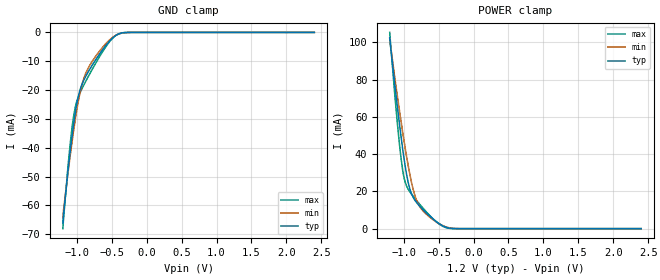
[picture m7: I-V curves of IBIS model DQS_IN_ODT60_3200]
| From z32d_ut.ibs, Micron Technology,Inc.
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| MODEL DQS_IN_ODT60_3200 (Data Strobe Input with 60ohm ODT, 1600-3200Mbps)
[Model]   DQS_IN_ODT60_3200
Model_type   Input
Vinl = 905.000mV
Vinh = 1015.000mV
|   typ   min   max
|C_comp   0.596pF   0.538pF   0.646pF
C_comp_power_clamp   0.298pF   0.269pF   0.323pF
C_comp_gnd_clamp   0.298pF   0.269pF   0.323pF
| Note: C_comp changes when the ODT circuit is enabled.
|[Model Spec]
| Dynamic Overshoot Parameters from DDR4 Specification
|D_overshoot_ampl_h   0.40   NA   NA
|D_overshoot_ampl_l   0.40   NA   NA
|D_overshoot_area_h   0.0800n   NA   NA
|D_overshoot_area_l   0.0800n   NA   NA
[Voltage Range]   1.2000V   1.1400V   1.2600V
| Junction Temperature (Ambient temp is 35C typ, 125C min, -40C max)
[Temperature Range]   50.0   140.0   -40.0
[Add Submodel]
| Submodel Name   Mode
60ohm_ODT_3200   Non-Driving
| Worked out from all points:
|   GND clamp passes 1 mA (typ) near -0.44 V on its own axis
|   POWER clamp passes 1 mA (typ) near -0.41 V on its own axis
[GND Clamp]
|   Voltage   I(typ)   I(min)   I(max)
-1.2V     -66.16mA   -64.28mA   -68.09mA
-1.135V   -50.09mA   -50.4mA    -48.84mA
-1.091V   -40.54mA   -42.05mA   -37.85mA
-1.047V   -32.06mA   -34.29mA   -29.28mA
-1.004V   -25.24mA   -27.37mA   -24.15mA
-960mV    -20.46mA   -21.61mA   -21.27mA
-916.4mV  -17.45mA   -17.25mA   -19.05mA
-840mV    -13.84mA   -12.54mA   -15.5mA
-643.6mV  -6.426mA   -5.55mA    -7.18mA
-458.2mV  -1.359mA   -1.253mA   -1.332mA
-250.9mV  -9.002uA   -25.19uA   1.741uA
2.4V      0A         0A         0A
[POWER Clamp]
|   Voltage   I(typ)   I(min)   I(max)
-1.2V     102.5mA    102mA      105.3mA
-1.135V   79.77mA    83.1mA     75.19mA
-1.08V    62.13mA    68.42mA    52.54mA
-1.036V   48.91mA    57.17mA    37.32mA
-992.7mV  37.04mA    46.51mA    27.02mA
-916.4mV  21.89mA    29.93mA    20mA
-861.8mV  16.57mA    20.7mA     17.26mA
-807.3mV  13.63mA    14.48mA    14.72mA
-709.1mV  9.665mA    8.958mA    10.4mA
-512.7mV  3.198mA    3.102mA    3.061mA
-250.9mV  21.9uA     63.81uA    -1.736uA
2.4V      0A         0A         0A
